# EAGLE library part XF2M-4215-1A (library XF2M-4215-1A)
FFC & FPC Connectors .5mm Rotary BackLock SMT Dual 42P Adhesv. Source: Datasheet
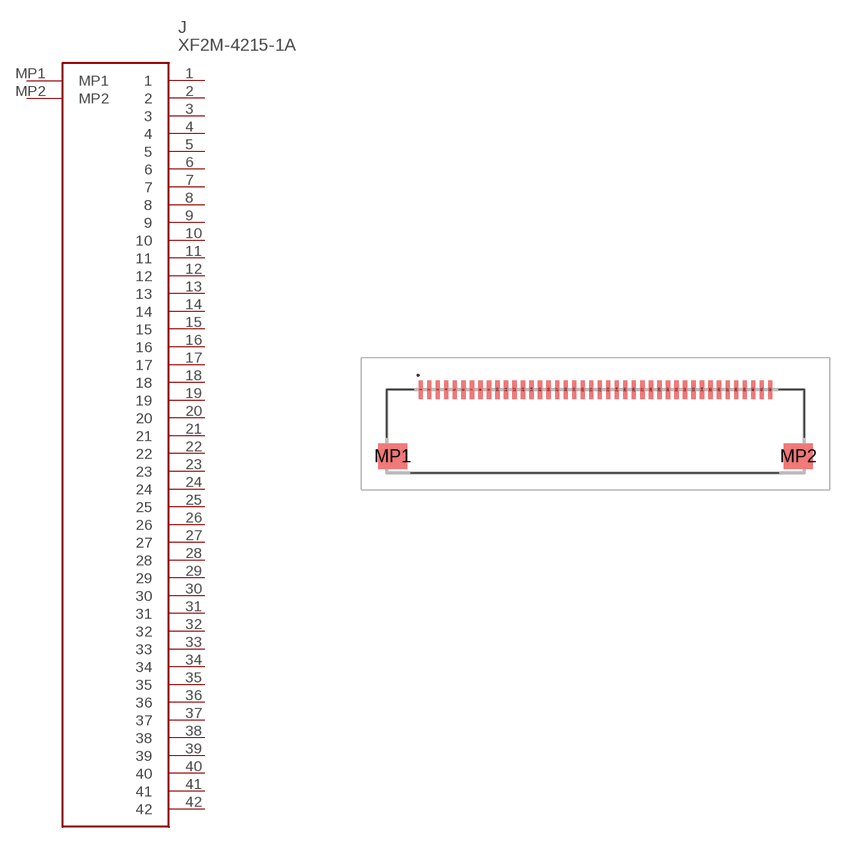
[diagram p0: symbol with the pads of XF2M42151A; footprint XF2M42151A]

Designator prefix J

## XF2M-4215-1A (Description: FFC & FPC Connectors .5mm Rotary BackLock SMT Dual 42P Adhesv.; Height: 3.2mm; Manufacturer_Name: Omron Electronics; Manufacturer_Part_Number: XF2M-4215-1A; Mouser_Part_Number: 653-XF2M-4215-1A; Mouser_Price-Stock: https://www.mouser.co.uk/ProductDetail/Omron-Electronics/XF2M-4215-1A?qs=WOBxwZpV8jU7WBv6l1ZdqA%3D%3D)  [XF2M42151A]
1  1
2  2
3  3
4  4
5  5
6  6
7  7
8  8
9  9
10  10
11  11
12  12
13  13
14  14
15  15
16  16
17  17
18  18
19  19
20  20
21  21
22  22
23  23
24  24
25  25
26  26
27  27
28  28
29  29
30  30
31  31
32  32
33  33
34  34
35  35
36  36
37  37
38  38
39  39
40  40
41  41
42  42
MP1  MP1
MP2  MP2

## Footprint XF2M42151A (pad centres in mm)
XF2M-4215-1A-1
smd 0.25 x 1.1: 1 -10,0; 2 -9.5,0; 3 -9,0; 4 -8.5,0; 5 -8,0; 6 -7.5,0; 7 -7,0; 8 -6.5,0; 9 -6,0; 10 -5.5,0; 11 -5,0; 12 -4.5,0; 13 -4,0; 14 -3.5,0; 15 -3,0; 16 -2.5,0; 17 -2,0; 18 -1.5,0; 19 -1,0; 20 -0.5,0; 21 0,0; 22 0.5,0; 23 1,0; 24 1.5,0; 25 2,0; 26 2.5,0; 27 3,0; 28 3.5,0; 29 4,0; 30 4.5,0; 31 5,0; 32 5.5,0; 33 6,0; 34 6.5,0; 35 7,0; 36 7.5,0; 37 8,0; 38 8.5,0; 39 9,0; 40 9.5,0; 41 10,0; 42 10.5,0
smd 1.7 x 1.5: MP1 -11.65,-3.9; MP2 12.15,-3.9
